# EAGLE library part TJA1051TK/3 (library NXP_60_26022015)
High-speed CAN transceiver The TJA1051 is a high-speed CAN transceiver that provides an interface between a Controller Area Network (CAN) protocol controller and the physical two-wire CAN bus. The transceiver is designed for high-speed (up to 1 Mbit/s) CAN applications in the automotive industry, providing differential transmit and receive capability to (a microcontroller with) a CAN protocol controller. The TJA1051 belongs to the third generation of high-speed CAN transceivers from NXP Semiconductors, offering significant improvements over first- and second-generation devices such as the TJA1050. It offers improved ElectroMagnetic Compatibility (EMC) and ElectroStatic Discharge (ESD) performance, and also features: Ideal passive behavior to the CAN bus when the supply voltage is off TJA1051T/3 and TJA1051TK/3 can be interfaced directly to microcontrollers with supply voltages from 3 V to 5 V These features make the TJA1051 an excellent choice for all types of HS-CAN networks, in nodes that do not require a standby mode with wake-up capability via the bus. AAL Eindhoven MK
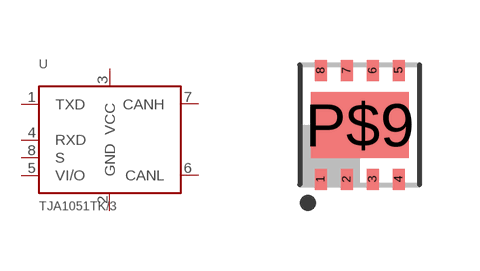
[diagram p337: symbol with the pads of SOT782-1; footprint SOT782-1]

Designator prefix U

## TJA1051TK/3  [SOT782-1]
1  TXD  out
2  GND
3  VCC
4  RXD
5  VI/O  pas
6  CANL
7  CANH
8  S  pwr

## Footprint SOT782-1 (pad centres in mm)
SOT782-1 HVSON8: plastic thermal enhanced very thin small outline package; no leads; 8 terminals; body 3 x 3 x 0.85 mm JEDEC: MO-229 IEC: -- JEITA: --
smd 0.3 x 0.525: 1 -0.975,-1.363; 2 -0.325,-1.363; 3 0.325,-1.363; 4 0.975,-1.363; 5 0.975,1.363; 6 0.325,1.363; 7 -0.325,1.363; 8 -0.975,1.363
smd 2.45 x 1.65: P$9 0,0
